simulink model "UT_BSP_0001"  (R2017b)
settings: Solver=FixedStepDiscrete  StartTime=0.0  StopTime=3  FixedStep=0.01  RelTol=1e-3  EnableMultiTasking=on
undefined symbols (not defined in the file): sigbuilder_block

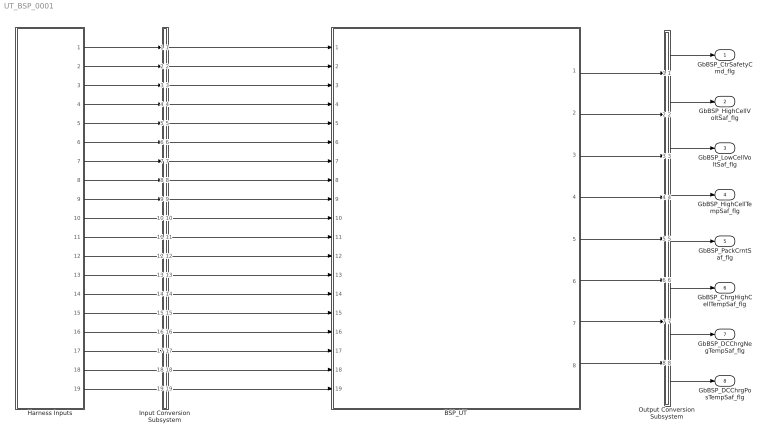
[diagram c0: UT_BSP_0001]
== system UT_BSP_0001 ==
  BSP_UT : ModelReference  ModelNameDialog=BSP_UT  SimulationMode=Normal  ModelReferenceVersion='M104C107'
  Harness Inputs : Subsystem  Tag=STV Subsys  LoadFcn=sigbuilder_block('load');  StartFcn=sigbuilder_block('start');  StopFcn=sigbuilder_block('stop');  ClipboardFcn=sigbuilder_block('clipboard');  mask(Sigbuilder block){tuvar=[0:10]}
      mask init:
      | if ~strcmp(get_param(bdroot(gcb),'SimulationStatus'),'stopped'),tuvar = sigbuilder_block('maskInit'); end
  Input Conversion Subsystem : Subsystem  Tag=__SLT_ICS__  Description=Signal spec. and routing
  Output Conversion Subsystem : Subsystem  Tag=__SLT_OCS__  Description=Signal spec. and routing
  GbBSP_CtrSafetyCmd_flg : Outport  OutDataTypeStr=boolean  PortDimensions=[1]
  GbBSP_HighCellVoltSaf_flg : Outport  Port=2  OutDataTypeStr=boolean  PortDimensions=[1]
  GbBSP_LowCellVoltSaf_flg : Outport  Port=3  OutDataTypeStr=boolean  PortDimensions=[1]
  GbBSP_HighCellTempSaf_flg : Outport  Port=4  OutDataTypeStr=boolean  PortDimensions=[1]
  GbBSP_PackCrntSaf_flg : Outport  Port=5  OutDataTypeStr=boolean  PortDimensions=[1]
  GbBSP_ChrgHighCellTempSaf_flg : Outport  Port=6  OutDataTypeStr=boolean  PortDimensions=[1]
  GbBSP_DCChrgNegTempSaf_flg : Outport  Port=7  OutDataTypeStr=boolean  PortDimensions=[1]
  GbBSP_DCChrgPosTempSaf_flg : Outport  Port=8  OutDataTypeStr=boolean  PortDimensions=[1]
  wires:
  Harness Inputs/1(GcCDP_MaxCellVolt_mV) -> Input Conversion Subsystem/1(Inport_1)
  Harness Inputs/2(GcCDP_MinCellVolt_mV) -> Input Conversion Subsystem/2(Inport_2)
  Harness Inputs/3(GcCDP_MaxCellTemp_C) -> Input Conversion Subsystem/3(Inport_3)
  Harness Inputs/4(GcCDP_MinCellTemp_C) -> Input Conversion Subsystem/4(Inport_4)
  Harness Inputs/5(GcHDP_PackCrnt_A) -> Input Conversion Subsystem/5(Inport_5)
  Harness Inputs/6(GbISP_TFHighCellTempSaf_flg) -> Input Conversion Subsystem/6(Inport_6)
  Harness Inputs/7(GbISP_TFLowCellVoltSaf_flg) -> Input Conversion Subsystem/7(Inport_7)
  Harness Inputs/8(GbISP_TFPackCrntSaf_flg) -> Input Conversion Subsystem/8(Inport_8)
  Harness Inputs/9(GbISP_TFHighCellVoltSaf_flg) -> Input Conversion Subsystem/9(Inport_9)
  Harness Inputs/10(GeCTC_CtrCtlConnMode_enum) -> Input Conversion Subsystem/10(Inport_10)
  Harness Inputs/11(GeUDS_CapSel_enum) -> Input Conversion Subsystem/11(Inport_11)
  Harness Inputs/12(GbLDP_DCChrgNegTempSTVFlt_flg) -> Input Conversion Subsystem/12(Inport_12)
  Harness Inputs/13(GbLDP_DCChrgNegTempSTGFlt_flg) -> Input Conversion Subsystem/13(Inport_13)
  Harness Inputs/14(GcLDP_ChrgTempNeg_C) -> Input Conversion Subsystem/14(Inport_14)
  Harness Inputs/15(GbLDP_DCChrgPosTempSTVFlt_flg) -> Input Conversion Subsystem/15(Inport_15)
  Harness Inputs/16(GbLDP_DCChrgPosTempSTGFlt_flg) -> Input Conversion Subsystem/16(Inport_16)
  Harness Inputs/17(GcLDP_ChrgTempPos_C) -> Input Conversion Subsystem/17(Inport_17)
  Harness Inputs/18(GbISP_TFDCChrgNegTempSaf_flg) -> Input Conversion Subsystem/18(Inport_18)
  Harness Inputs/19(GbISP_TFDCChrgPosTempSaf_flg) -> Input Conversion Subsystem/19(Inport_19)
  Output Conversion Subsystem/1(Outport_1) -> GbBSP_CtrSafetyCmd_flg/1
  Output Conversion Subsystem/2(Outport_2) -> GbBSP_HighCellVoltSaf_flg/1
  Output Conversion Subsystem/3(Outport_3) -> GbBSP_LowCellVoltSaf_flg/1
  Output Conversion Subsystem/4(Outport_4) -> GbBSP_HighCellTempSaf_flg/1
  Output Conversion Subsystem/5(Outport_5) -> GbBSP_PackCrntSaf_flg/1
  Output Conversion Subsystem/6(Outport_6) -> GbBSP_ChrgHighCellTempSaf_flg/1
  Output Conversion Subsystem/7(Outport_7) -> GbBSP_DCChrgNegTempSaf_flg/1
  Output Conversion Subsystem/8(Outport_8) -> GbBSP_DCChrgPosTempSaf_flg/1
  Input Conversion Subsystem/1(Outport_1) -> BSP_UT/1
  Input Conversion Subsystem/2(Outport_2) -> BSP_UT/2
  Input Conversion Subsystem/3(Outport_3) -> BSP_UT/3
  Input Conversion Subsystem/4(Outport_4) -> BSP_UT/4
  Input Conversion Subsystem/5(Outport_5) -> BSP_UT/5
  Input Conversion Subsystem/6(Outport_6) -> BSP_UT/6
  Input Conversion Subsystem/7(Outport_7) -> BSP_UT/7
  Input Conversion Subsystem/8(Outport_8) -> BSP_UT/8
  Input Conversion Subsystem/9(Outport_9) -> BSP_UT/9
  Input Conversion Subsystem/10(Outport_10) -> BSP_UT/10
  Input Conversion Subsystem/11(Outport_11) -> BSP_UT/11
  Input Conversion Subsystem/12(Outport_12) -> BSP_UT/12
  Input Conversion Subsystem/13(Outport_13) -> BSP_UT/13
  Input Conversion Subsystem/14(Outport_14) -> BSP_UT/14
  Input Conversion Subsystem/15(Outport_15) -> BSP_UT/15
  Input Conversion Subsystem/16(Outport_16) -> BSP_UT/16
  Input Conversion Subsystem/17(Outport_17) -> BSP_UT/17
  Input Conversion Subsystem/18(Outport_18) -> BSP_UT/18
  Input Conversion Subsystem/19(Outport_19) -> BSP_UT/19
  BSP_UT/1 -> Output Conversion Subsystem/1(Inport_1)
  BSP_UT/2 -> Output Conversion Subsystem/2(Inport_2)
  BSP_UT/3 -> Output Conversion Subsystem/3(Inport_3)
  BSP_UT/4 -> Output Conversion Subsystem/4(Inport_4)
  BSP_UT/5 -> Output Conversion Subsystem/5(Inport_5)
  BSP_UT/6 -> Output Conversion Subsystem/6(Inport_6)
  BSP_UT/7 -> Output Conversion Subsystem/7(Inport_7)
  BSP_UT/8 -> Output Conversion Subsystem/8(Inport_8)

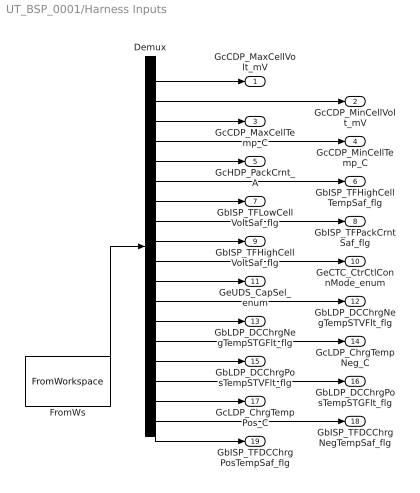
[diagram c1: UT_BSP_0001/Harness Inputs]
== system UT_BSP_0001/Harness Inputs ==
  Demux : Demux  Tag=STV Demux  Outputs=19
  FromWs : FromWorkspace  Tag=STV FromWs  VariableName=tuvar  SampleTime=0
  GcCDP_MaxCellVolt_mV : Outport  Tag=STV Outport
  GcCDP_MinCellVolt_mV : Outport  Tag=STV Outport  Port=2
  GcCDP_MaxCellTemp_C : Outport  Tag=STV Outport  Port=3
  GcCDP_MinCellTemp_C : Outport  Tag=STV Outport  Port=4
  GcHDP_PackCrnt_A : Outport  Tag=STV Outport  Port=5
  GbISP_TFHighCellTempSaf_flg : Outport  Tag=STV Outport  Port=6
  GbISP_TFLowCellVoltSaf_flg : Outport  Tag=STV Outport  Port=7
  GbISP_TFPackCrntSaf_flg : Outport  Tag=STV Outport  Port=8
  GbISP_TFHighCellVoltSaf_flg : Outport  Tag=STV Outport  Port=9
  GeCTC_CtrCtlConnMode_enum : Outport  Tag=STV Outport  Port=10
  GeUDS_CapSel_enum : Outport  Tag=STV Outport  Port=11
  GbLDP_DCChrgNegTempSTVFlt_flg : Outport  Tag=STV Outport  Port=12
  GbLDP_DCChrgNegTempSTGFlt_flg : Outport  Tag=STV Outport  Port=13
  GcLDP_ChrgTempNeg_C : Outport  Tag=STV Outport  Port=14
  GbLDP_DCChrgPosTempSTVFlt_flg : Outport  Tag=STV Outport  Port=15
  GbLDP_DCChrgPosTempSTGFlt_flg : Outport  Tag=STV Outport  Port=16
  GcLDP_ChrgTempPos_C : Outport  Tag=STV Outport  Port=17
  GbISP_TFDCChrgNegTempSaf_flg : Outport  Tag=STV Outport  Port=18
  GbISP_TFDCChrgPosTempSaf_flg : Outport  Tag=STV Outport  Port=19
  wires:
  FromWs/1 -> Demux/1
  Demux/1 -> GcCDP_MaxCellVolt_mV/1
  Demux/2 -> GcCDP_MinCellVolt_mV/1
  Demux/3 -> GcCDP_MaxCellTemp_C/1
  Demux/4 -> GcCDP_MinCellTemp_C/1
  Demux/5 -> GcHDP_PackCrnt_A/1
  Demux/6 -> GbISP_TFHighCellTempSaf_flg/1
  Demux/7 -> GbISP_TFLowCellVoltSaf_flg/1
  Demux/8 -> GbISP_TFPackCrntSaf_flg/1
  Demux/9 -> GbISP_TFHighCellVoltSaf_flg/1
  Demux/10 -> GeCTC_CtrCtlConnMode_enum/1
  Demux/11 -> GeUDS_CapSel_enum/1
  Demux/12 -> GbLDP_DCChrgNegTempSTVFlt_flg/1
  Demux/13 -> GbLDP_DCChrgNegTempSTGFlt_flg/1
  Demux/14 -> GcLDP_ChrgTempNeg_C/1
  Demux/15 -> GbLDP_DCChrgPosTempSTVFlt_flg/1
  Demux/16 -> GbLDP_DCChrgPosTempSTGFlt_flg/1
  Demux/17 -> GcLDP_ChrgTempPos_C/1
  Demux/18 -> GbISP_TFDCChrgNegTempSaf_flg/1
  Demux/19 -> GbISP_TFDCChrgPosTempSaf_flg/1

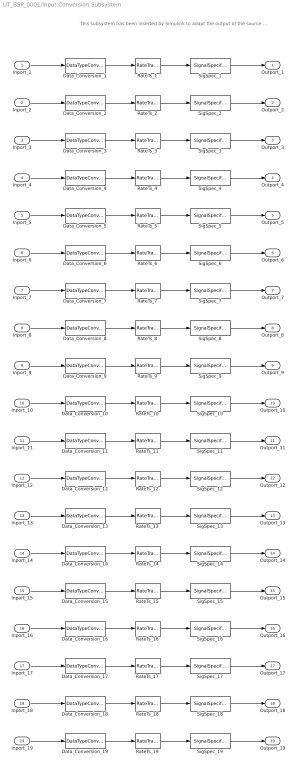
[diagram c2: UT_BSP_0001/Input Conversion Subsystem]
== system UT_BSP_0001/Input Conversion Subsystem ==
  note: This subsystem has been inserted by Simulink to adapt the output of the source blocks to the interface required by the harnessed component. Modifying the contents of this subsystem may result in compilation and simulation failure.
  Inport_1 : Inport
  Inport_2 : Inport  Port=2
  Inport_3 : Inport  Port=3
  Inport_4 : Inport  Port=4
  Inport_5 : Inport  Port=5
  Inport_6 : Inport  Port=6
  Inport_7 : Inport  Port=7
  Inport_8 : Inport  Port=8
  Inport_9 : Inport  Port=9
  Inport_10 : Inport  Port=10
  Inport_11 : Inport  Port=11
  Inport_12 : Inport  Port=12
  Inport_13 : Inport  Port=13
  Inport_14 : Inport  Port=14
  Inport_15 : Inport  Port=15
  Inport_16 : Inport  Port=16
  Inport_17 : Inport  Port=17
  Inport_18 : Inport  Port=18
  Inport_19 : Inport  Port=19
  Data_Conversion_1 : DataTypeConversion  OutDataTypeStr=uint16
  Data_Conversion_10 : DataTypeConversion  OutDataTypeStr=uint8
  Data_Conversion_11 : DataTypeConversion  OutDataTypeStr=uint8
  Data_Conversion_{6..9,12..13,15..16,18..19} (10 alike) : DataTypeConversion  OutDataTypeStr=boolean
  Data_Conversion_{3..5,14,17} (5 alike) : DataTypeConversion  OutDataTypeStr=single
  Data_Conversion_2 : DataTypeConversion  OutDataTypeStr=uint16
  RateTs_{1..19} (19 alike) : RateTransition  OutPortSampleTime=0.01
  SigSpec_1 : SignalSpecification  OutDataTypeStr=uint16  Unit=mV  Dimensions=[1]  SampleTime=0.01
  SigSpec_10 : SignalSpecification  OutDataTypeStr=uint8  Unit=enum  Dimensions=[1]  SampleTime=0.01
  SigSpec_11 : SignalSpecification  OutDataTypeStr=uint8  Unit=enum  Dimensions=[1]  SampleTime=0.01
  SigSpec_{6..9,12..13,15..16,18..19} (10 alike) : SignalSpecification  OutDataTypeStr=boolean  Unit=flag  Dimensions=[1]  SampleTime=0.01
  SigSpec_{3..4,14,17} (4 alike) : SignalSpecification  OutDataTypeStr=single  Unit=C  Dimensions=[1]  SampleTime=0.01
  SigSpec_2 : SignalSpecification  OutDataTypeStr=uint16  Unit=mV  Dimensions=[1]  SampleTime=0.01
  SigSpec_5 : SignalSpecification  OutDataTypeStr=single  Unit=A  Dimensions=[1]  SampleTime=0.01
  Outport_1 : Outport
  Outport_2 : Outport  Port=2
  Outport_3 : Outport  Port=3
  Outport_4 : Outport  Port=4
  Outport_5 : Outport  Port=5
  Outport_6 : Outport  Port=6
  Outport_7 : Outport  Port=7
  Outport_8 : Outport  Port=8
  Outport_9 : Outport  Port=9
  Outport_10 : Outport  Port=10
  Outport_11 : Outport  Port=11
  Outport_12 : Outport  Port=12
  Outport_13 : Outport  Port=13
  Outport_14 : Outport  Port=14
  Outport_15 : Outport  Port=15
  Outport_16 : Outport  Port=16
  Outport_17 : Outport  Port=17
  Outport_18 : Outport  Port=18
  Outport_19 : Outport  Port=19
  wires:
  SigSpec_1/1 -> Outport_1/1
  RateTs_1/1 -> SigSpec_1/1
  Data_Conversion_1/1 -> RateTs_1/1
  Inport_1/1 -> Data_Conversion_1/1
  SigSpec_2/1 -> Outport_2/1
  RateTs_2/1 -> SigSpec_2/1
  Data_Conversion_2/1 -> RateTs_2/1
  Inport_2/1 -> Data_Conversion_2/1
  SigSpec_3/1 -> Outport_3/1
  RateTs_3/1 -> SigSpec_3/1
  Data_Conversion_3/1 -> RateTs_3/1
  Inport_3/1 -> Data_Conversion_3/1
  SigSpec_4/1 -> Outport_4/1
  RateTs_4/1 -> SigSpec_4/1
  Data_Conversion_4/1 -> RateTs_4/1
  Inport_4/1 -> Data_Conversion_4/1
  SigSpec_5/1 -> Outport_5/1
  RateTs_5/1 -> SigSpec_5/1
  Data_Conversion_5/1 -> RateTs_5/1
  Inport_5/1 -> Data_Conversion_5/1
  SigSpec_6/1 -> Outport_6/1
  RateTs_6/1 -> SigSpec_6/1
  Data_Conversion_6/1 -> RateTs_6/1
  Inport_6/1 -> Data_Conversion_6/1
  SigSpec_7/1 -> Outport_7/1
  RateTs_7/1 -> SigSpec_7/1
  Data_Conversion_7/1 -> RateTs_7/1
  Inport_7/1 -> Data_Conversion_7/1
  SigSpec_8/1 -> Outport_8/1
  RateTs_8/1 -> SigSpec_8/1
  Data_Conversion_8/1 -> RateTs_8/1
  Inport_8/1 -> Data_Conversion_8/1
  SigSpec_9/1 -> Outport_9/1
  RateTs_9/1 -> SigSpec_9/1
  Data_Conversion_9/1 -> RateTs_9/1
  Inport_9/1 -> Data_Conversion_9/1
  SigSpec_10/1 -> Outport_10/1
  RateTs_10/1 -> SigSpec_10/1
  Data_Conversion_10/1 -> RateTs_10/1
  Inport_10/1 -> Data_Conversion_10/1
  SigSpec_11/1 -> Outport_11/1
  RateTs_11/1 -> SigSpec_11/1
  Data_Conversion_11/1 -> RateTs_11/1
  Inport_11/1 -> Data_Conversion_11/1
  SigSpec_12/1 -> Outport_12/1
  RateTs_12/1 -> SigSpec_12/1
  Data_Conversion_12/1 -> RateTs_12/1
  Inport_12/1 -> Data_Conversion_12/1
  SigSpec_13/1 -> Outport_13/1
  RateTs_13/1 -> SigSpec_13/1
  Data_Conversion_13/1 -> RateTs_13/1
  Inport_13/1 -> Data_Conversion_13/1
  SigSpec_14/1 -> Outport_14/1
  RateTs_14/1 -> SigSpec_14/1
  Data_Conversion_14/1 -> RateTs_14/1
  Inport_14/1 -> Data_Conversion_14/1
  SigSpec_15/1 -> Outport_15/1
  RateTs_15/1 -> SigSpec_15/1
  Data_Conversion_15/1 -> RateTs_15/1
  Inport_15/1 -> Data_Conversion_15/1
  SigSpec_16/1 -> Outport_16/1
  RateTs_16/1 -> SigSpec_16/1
  Data_Conversion_16/1 -> RateTs_16/1
  Inport_16/1 -> Data_Conversion_16/1
  SigSpec_17/1 -> Outport_17/1
  RateTs_17/1 -> SigSpec_17/1
  Data_Conversion_17/1 -> RateTs_17/1
  Inport_17/1 -> Data_Conversion_17/1
  SigSpec_18/1 -> Outport_18/1
  RateTs_18/1 -> SigSpec_18/1
  Data_Conversion_18/1 -> RateTs_18/1
  Inport_18/1 -> Data_Conversion_18/1
  SigSpec_19/1 -> Outport_19/1
  RateTs_19/1 -> SigSpec_19/1
  Data_Conversion_19/1 -> RateTs_19/1
  Inport_19/1 -> Data_Conversion_19/1

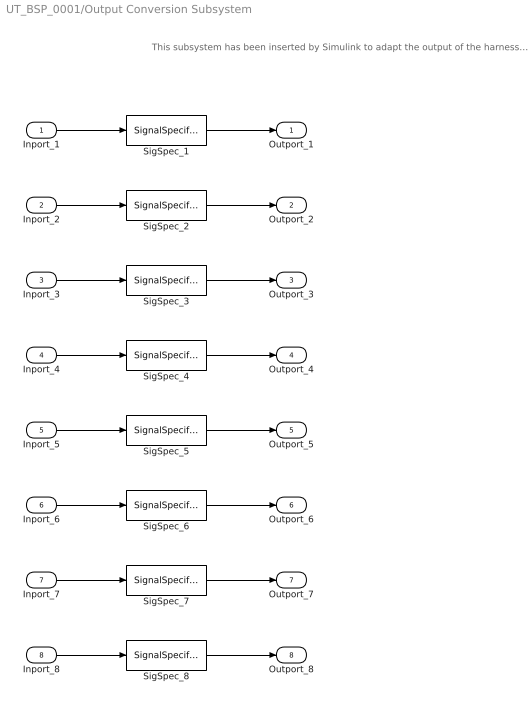
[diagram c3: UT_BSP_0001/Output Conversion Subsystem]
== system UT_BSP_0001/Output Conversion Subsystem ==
  note: This subsystem has been inserted by Simulink to adapt the output of the harnessed component to the interface required by the sink blocks. Modifying the contents of this subsystem may result in compilation and simulation failure.
  Inport_1 : Inport
  Inport_2 : Inport  Port=2
  Inport_3 : Inport  Port=3
  Inport_4 : Inport  Port=4
  Inport_5 : Inport  Port=5
  Inport_6 : Inport  Port=6
  Inport_7 : Inport  Port=7
  Inport_8 : Inport  Port=8
  SigSpec_{1..8} (8 alike) : SignalSpecification  OutDataTypeStr=boolean  Unit=flag  Dimensions=[1]  SampleTime=0.01
  Outport_1 : Outport
  Outport_2 : Outport  Port=2
  Outport_3 : Outport  Port=3
  Outport_4 : Outport  Port=4
  Outport_5 : Outport  Port=5
  Outport_6 : Outport  Port=6
  Outport_7 : Outport  Port=7
  Outport_8 : Outport  Port=8
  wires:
  Inport_1/1 -> SigSpec_1/1
  SigSpec_1/1 -> Outport_1/1
  Inport_2/1 -> SigSpec_2/1
  SigSpec_2/1 -> Outport_2/1
  Inport_3/1 -> SigSpec_3/1
  SigSpec_3/1 -> Outport_3/1
  Inport_4/1 -> SigSpec_4/1
  SigSpec_4/1 -> Outport_4/1
  Inport_5/1 -> SigSpec_5/1
  SigSpec_5/1 -> Outport_5/1
  Inport_6/1 -> SigSpec_6/1
  SigSpec_6/1 -> Outport_6/1
  Inport_7/1 -> SigSpec_7/1
  SigSpec_7/1 -> Outport_7/1
  Inport_8/1 -> SigSpec_8/1
  SigSpec_8/1 -> Outport_8/1
